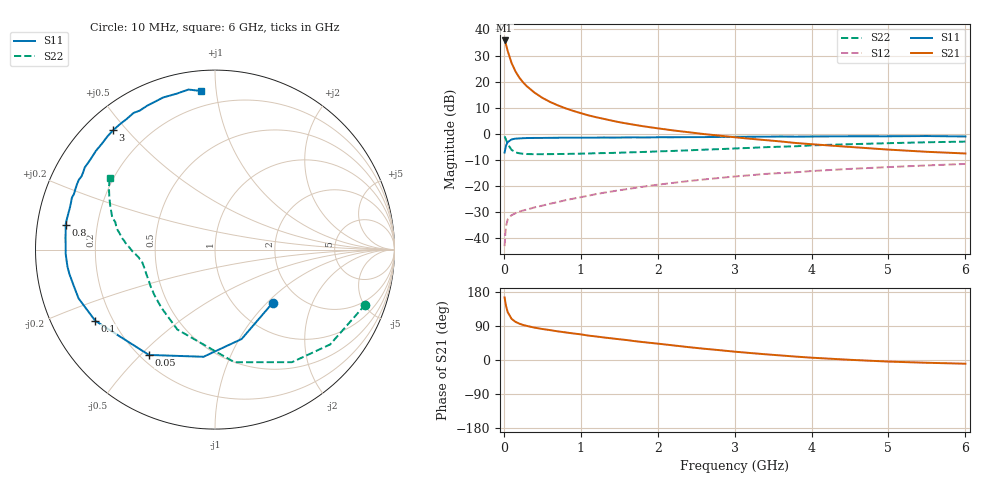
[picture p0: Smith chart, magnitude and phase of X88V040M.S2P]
! SIEMENS Small Signal Semiconductors
! BFP136W
! Si NPN RF Bipolar Junction Transistor in SOT343
! VCE = 8 V  IC = 40 mA
! Common Emitter S-Parameters:  September  1994
# GHz  S  MA  R  50
!  f  S11  S21  S12  S22
! GHz  MAG  ANG  MAG  ANG  MAG  ANG  MAG  ANG
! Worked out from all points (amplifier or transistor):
!   40 points, 10 MHz to 6 GHz, reference 50 ohm
!   highest |S21| = 35.8 dB at 10 MHz (marker M1)
!   |S21| within 3 dB of that: start of sweep to 40.96 MHz
!   unconditionally stable (mu >= 1): 861.9 MHz to 2.903 GHz
!   at 200 MHz: K = 0.47, MSG = 25.7 dB, |S12| = -29.9 dB
!   at 1.5 GHz: K = 1.11, MAG = 11.0 dB, |S12| = -21.7 dB
!   at 6 GHz: K = 0.95, MSG = 2.0 dB, |S12| = -11.6 dB
!   S11 on the Smith chart (normalised r, x): 10 MHz: 1.48, -1.08; 50 MHz: 0.23, -0.53; 100 MHz: 0.14, -0.27; 800 MHz: 0.09, +0.08; 3 GHz: 0.08, +0.46; 6 GHz: 0.11, +0.91
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0.01  0.4373 -42.5  61.49 165.2  0.007 73.9  0.8918 -20.1
0.02  0.5197 -73.4  55.75 152.0  0.0124 64.6  0.8311 -39.5
0.03  0.6005 -96.1  50.19 141.4  0.0173 55.7  0.76 -55.6
0.05  0.6928 -122.1  38.71 126.4  0.0228 43.4  0.6367 -80.2
0.1  0.7763 -149.3  22.86 108.8  0.0275 33.4  0.4923 -115.2
0.15  0.8073 -160.3  15.83 100.8  0.0299 31.5  0.4408 -132.6
0.2  0.8134 -166.2  11.99 96.0  0.0321 31.4  0.4224 -142.9
0.25  0.8225 -170.5  9.69 92.4  0.0338 32.4  0.4141 -149.5
0.3  0.8275 -173.4  8.115 89.9  0.0352 34.1  0.4082 -154.1
0.4  0.8323 -178.4  6.131 85.4  0.0388 36.8  0.4062 -160.1
0.5  0.8326 178.1  4.892 81.8  0.0419 39.5  0.4061 -164.0
0.6  0.8356 175.5  4.082 78.9  0.0455 41.6  0.4071 -166.3
0.7  0.8386 172.6  3.519 75.6  0.049 44.3  0.409 -168.0
0.8  0.8438 170.6  3.08 72.9  0.0532 46.1  0.4107 -169.5
1.1  0.8417 163.8  2.25 64.4  0.065 49.8  0.4193 -172.4
1.5  0.8469 156.9  1.667 54.8  0.0826 52.3  0.4333 -175.1
2.2  0.8566 144.3  1.16 38.6  0.1144 51.3  0.4687 179.8
3  0.8744 130.5  0.858 22.0  0.1516 46.5  0.5224 172.9
3.2  0.8767 127.2  0.802 18.5  0.1602 45.0  0.5362 170.7
4.5  0.8954 108.8  0.559 0.5  0.2122 34.9  0.6308 157.6
5.5  0.904 99.4  0.451 -7.3  0.2471 26.7  0.6873 149.3
6  0.887 95.1  0.419 -9.8  0.2641 22.4  0.7073 145.8
